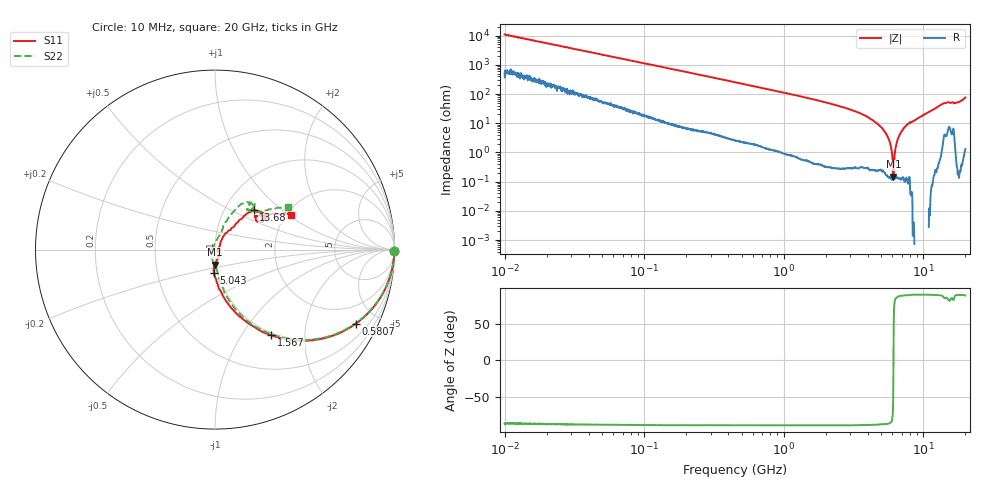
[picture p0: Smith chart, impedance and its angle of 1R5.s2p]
!Keysight Technologies,P5008B,MY61100088,A.16.20.02
!Date: Friday, August 30, 2024 11:00:47
!Correction: S11(C  2-Port  )
!S21(C  2-Port  )
!S12(C  2-Port  )
!S22(C  2-Port  )
!S2P File: Measurements: S11, S21, S12, S22:Log Frequency Sweep
# Hz S  dB  R 50
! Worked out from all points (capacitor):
!   1601 points, 10 MHz to 20 GHz, reference 50 ohm
!   read as one part in series: C = 1.46 pF near 10.39 MHz
!   lowest |Z| = 149 mohm at 6.099 GHz (marker M1)
!   series resonance near 6.106 GHz, so ESL is about 470 pH
!   S11 on the Smith chart (normalised r, x): 10 MHz: open; 580.7 MHz: 0.99, -3.82; 1.567 GHz: 0.96, -1.37; 5.043 GHz: 0.95, -0.25; 13.68 GHz: 1.36, +0.66; 20 GHz: 2.11, +1.05
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1e7  0.00 -0.5  -40.77 86.7  -40.75 86.9  -0.01 -0.5
3.555162e7  -0.01 -1.9  -29.88 86.4  -29.89 86.4  -0.01 -1.9
1.263918e8  -0.07 -6.6  -19.09 82.7  -19.10 82.7  -0.07 -6.5
4.472136e8  -0.66 -22.0  -8.76 67.5  -8.77 67.6  -0.65 -21.8
5.807482e8  -1.04 -27.7  -6.88 61.9  -6.89 61.9  -1.05 -27.4
9.933977e8  -2.52 -42.4  -3.64 47.4  -3.64 47.4  -2.53 -42.0
1.567418e9  -4.86 -56.7  -1.75 33.3  -1.76 33.2  -4.86 -56.0
1.589917e9  -4.95 -57.2  -1.71 32.8  -1.71 32.8  -4.95 -56.5
3.151135e9  -10.75 -78.1  -0.40 13.0  -0.41 13.0  -10.71 -74.6
5.043341e9  -17.66 -93.1  -0.08 0.4  -0.09 0.4  -17.68 -83.2
5.652411e9  -19.81 -93.8  -0.04 -2.6  -0.05 -2.6  -20.00 -88.1
6.098795e9  -21.61 -89.4  -0.02 -4.6  -0.02 -4.6  -21.94 -94.8
6.933443e9  -26.35 -68.4  0.01 -8.1  0.00 -8.1  -27.40 -119.9
8.344716e9  -35.96 -27.7  0.03 -13.4  0.02 -13.4  -40.33 -172.7
8.545299e9  -36.90 -26.3  0.03 -14.1  0.02 -14.2  -41.49 -179.8
8.961046e9  -34.03 10.3  0.03 -15.6  0.03 -15.7  -36.62 124.3
9.761022e9  -27.92 45.8  0.03 -18.6  0.03 -18.7  -28.69 88.2
1.043228e10  -23.12 56.3  0.02 -21.1  0.02 -21.2  -23.45 75.6
1.367661e10  -10.24 45.7  -0.45 -34.4  -0.45 -34.5  -10.32 57.9
1.599787e10  -9.64 34.2  -0.76 -38.9  -0.77 -39.0  -9.75 52.5
1.776035e10  -10.78 39.2  -0.34 -45.6  -0.35 -45.7  -10.75 47.6
2e10  -6.62 24.7  -1.13 -60.7  -1.13 -60.8  -6.53 30.4
